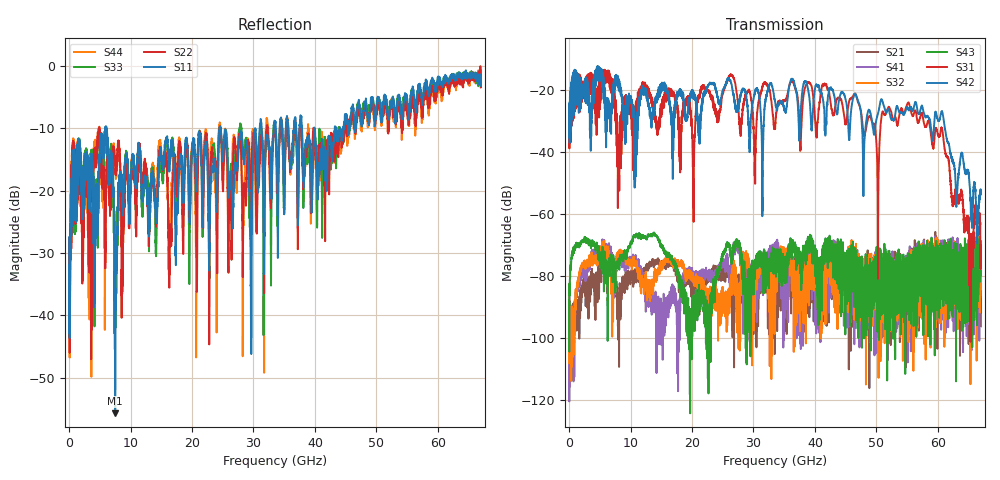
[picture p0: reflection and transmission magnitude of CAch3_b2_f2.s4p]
!Agilent Technologies,N5247A,US51170199,A.09.90.13
!Agilent N5247A: A.09.90.13
!Date: Thursday, October 18, 2018 09:45:05
!Correction: S11(Full 4 Port(1,2,3,4))
!S12(Full 4 Port(1,2,3,4))
!S13(Full 4 Port(1,2,3,4))
!S14(Full 4 Port(1,2,3,4))
!S21(Full 4 Port(1,2,3,4))
!S22(Full 4 Port(1,2,3,4))
!S23(Full 4 Port(1,2,3,4))
!S24(Full 4 Port(1,2,3,4))
!S31(Full 4 Port(1,2,3,4))
!S32(Full 4 Port(1,2,3,4))
!S33(Full 4 Port(1,2,3,4))
!S34(Full 4 Port(1,2,3,4))
!S41(Full 4 Port(1,2,3,4))
!S42(Full 4 Port(1,2,3,4))
!S43(Full 4 Port(1,2,3,4))
!S44(Full 4 Port(1,2,3,4))
!S4P File: Measurements: <S11,S12,S13,S14>,
!<S21,S22,S23,S24>,
!<S31,S32,S33,S34>,
!<S41,S42,S43,S44>:
# Hz S  dB  R 50
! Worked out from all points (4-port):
!   6701 points, 10 MHz to 67 GHz, reference 50 ohm
!   strongest paths, dB at 10 MHz, 16.76 GHz, 33.51 GHz, 50.25 GHz, 67 GHz:
!     S42: -30.0, -33.4, -23.7, -27.7, -52.8
!     S31: -30.3, -21.3, -32.0, -59.5, -72.5
!     S43: -88.0, -74.4, -73.6, -80.4, -72.3
!     S32: -83.0, -76.5, -80.3, -79.0, -72.2
!     S41: -95.3, -85.5, -70.6, -83.4, -83.2
!     S21: -83.3, -75.8, -86.1, -79.4, -96.3
!   lowest |S11| = -55.7 dB at 7.509 GHz (marker M1), VSWR 1.00, Z = 49.9 + j0.14 ohm
!   |S11| at or under -10 dB: start of sweep to 5.92 GHz; 6.063 GHz to 24.48 GHz (18.42 GHz wide, 121 % of centre); 24.67 GHz to 31.02 GHz (6.352 GHz wide, 22.8 % of centre)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
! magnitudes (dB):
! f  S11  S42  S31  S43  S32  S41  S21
! 10 MHz  -27.5  -30.0  -30.3  -88.0  -83.0  -95.3  -83.3
! 5.989 GHz  -9.7  -23.0  -13.9  -77.9  -73.7  -73.3  -77.7
! 7.509 GHz  -55.7  -17.5  -23.3  -83.3  -75.5  -76.9  -84.8
! 41.57 GHz  -16.6  -31.1  -18.0  -70.2  -74.5  -81.4  -84.1
! 50.25 GHz  -5.3  -27.7  -59.5  -80.4  -79.0  -83.4  -79.4
! 55.19 GHz  -6.8  -26.3  -24.1  -74.6  -89.6  -82.3  -82.7
! 67 GHz  -3.2  -52.8  -72.5  -72.3  -72.2  -83.2  -96.3
